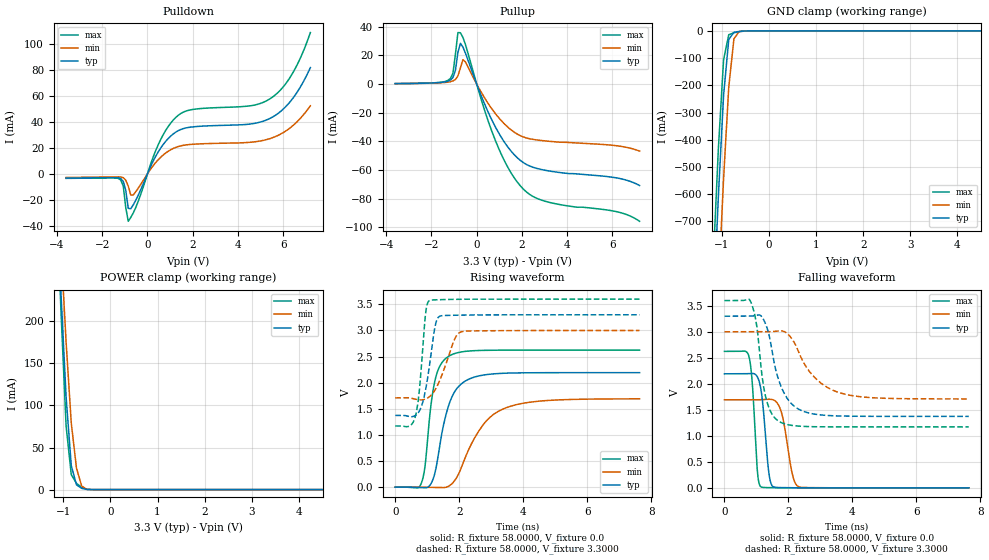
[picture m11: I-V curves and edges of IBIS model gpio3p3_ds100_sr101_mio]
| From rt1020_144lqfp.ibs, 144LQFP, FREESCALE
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[Model] gpio3p3_ds100_sr101_mio
|   Model gpio3p3_ds100_sr101_mio
| This model was characterised for following simulation conditions:
| External (pad) voltage:
|   - Typ: 3.3V,   - Min: 3.0V,   - Max: 3.6V
| Library cells for typ/min/max conditions are connected as defined below:
|  pad - External Pad
|  ipp_do - Core Input
|  ipp_obe - Output Buffer Enable
|  esd_boost - ovdd
|  ipp_dse0 - vssi
|  ipp_dse1 - vssi
|  ipp_dse2 - vddi
|  ipp_fsel0 - vddi
|  ipp_fsel1 - vssi
|  ipp_ina - ipp_ina
|  ipp_ind - ipp_ind
|  ipp_pwr_stable - vddi
|  ipp_sre - vddi
|  ovdd - ovdd
|  ovss - ovss
|  vddi - vddi
|  vssi - vssi
| All other pins connected to ground
Model_type I/O
Polarity   Non-Inverting
Enable   Active-High
Vinl =   0.9900V
Vinh =   2.3100V
Vmeas =  1.6500V
Cref =   0.0F
Rref =   58.0000
Vref =   1.6500V
C_comp   1.2178pF   1.1833pF   1.2636pF
|C_comp_pullup   0.6042pF   0.6189pF   0.5908pF
|C_comp_pulldown   0.5474pF   0.5788pF   0.5258pF
[Model Spec]
| variable   typ   min   max
Vinh   2.3100V   2.1000V   2.5200V
Vinl   0.9900V   0.9000V   1.0800V
S_overshoot_high   3.3000V   3.0000V   3.6000V
S_overshoot_low   0.0V   0.0V   0.0V
Vmeas   1.6500V   1.5000V   1.8000V
Vref   1.6500V   1.5000V   1.8000V
Cref   0.0F   0.0F   0.0F
Rref   58.0000   58.0000   58.0000
[Temperature Range]   25.0000   0.1050k   -20.0000
[Voltage Range]   3.3000V   3.0000V   3.6000V
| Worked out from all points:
|   slope of the pulldown table from 0 to 0.495 V, typ, clamps not added: 28.5 ohm
|   slope of the pullup table from 0 to 0.495 V, typ, clamps not added: 25.7 ohm
|   GND clamp passes 1 mA (typ) near -0.54 V on its own axis
|   POWER clamp passes 1 mA (typ) near -0.57 V on its own axis
|   rising waveform, R_fixture 58.0000, V_fixture 0.0: 20-80 % time 494ps typ, 946ps min, 310ps max; typ from 0 V to 2.19 V
|   rising waveform, R_fixture 58.0000, V_fixture 3.3000: 20-80 % time 287ps typ, 458ps min, 198ps max; typ from 1.37 V to 3.3 V
|   falling waveform, R_fixture 58.0000, V_fixture 0.0: 20-80 % time 187ps typ, 274ps min, 146ps max; typ from 2.19 V to 0 V
|   falling waveform, R_fixture 58.0000, V_fixture 3.3000: 20-80 % time 517ps typ, 894ps min, 318ps max; typ from 3.3 V to 1.37 V
[Pulldown]
|Voltage   I(typ)   I(min)   I(max)
-3.6V     -3.29mA    -2.84mA    -3.51mA
-1.18V    -3.645mA   -2.421mA   -4.835mA
-1.07V    -5.921mA   -3.024mA   -9.452mA
-960mV    -12.77mA   -4.911mA   -25.98mA
-850mV    -26.55mA   -9.409mA   -36.48mA
-630mV    -23.88mA   -16.25mA   -30.12mA
470mV     16.68mA    10.72mA    22.13mA
1.24V     31.86mA    20.19mA    43.07mA
1.9V      35.79mA    22.52mA    49.06mA
5.42V     42.57mA    27.03mA    57.6mA
6.3V      55.19mA    35.19mA    73.91mA
7.2V      81.51mA    52.18mA    108.4mA
[Pullup]
|Voltage   I(typ)   I(min)   I(max)
-3.6V     330uA      290uA      330uA
-1.27V    2.011mA    1.347mA    2.56mA
-1.05V    4.628mA    2.191mA    7.616mA
-940mV    9.591mA    3.262mA    21.02mA
-830mV    22.24mA    5.683mA    36mA
-720mV    28.46mA    11.34mA    35.87mA
-610mV    25.92mA    17.01mA    32.61mA
-500mV    21.74mA    15.5mA     27.75mA
820mV     -29.79mA   -20.52mA   -39.2mA
2.03V     -54.53mA   -36.77mA   -72.89mA
3.02V     -60.23mA   -39.71mA   -81.88mA
7.2V      -70.9mA    -46.86mA   -95.92mA
[GND_clamp]
|Voltage   I(typ)   I(min)   I(max)
-3.6V     -10.99A    -11.14A    -10.93A
-1.18V    -1.033A    -1.378A    -850.8mA
-1.07V    -607mA     -947.1mA   -431.4mA
-960mV    -236.8mA   -543mA     -106.4mA
-850mV    -31.63mA   -206.7mA   -14.18mA
-740mV    -5.424mA   -29mA      -7.092mA
-630mV    -2.275mA   -2.653mA   -3.283mA
-410mV    -62.05uA   -83.52uA   -82.05uA
7.2V      0A         0A         0A
[POWER_clamp]
|Voltage   I(typ)   I(min)   I(max)
-3.6V     3.491A     3.319A     3.949A
-1.16V    368.2mA    410.8mA    372.9mA
-1.05V    234.5mA    290.2mA    214.3mA
-940mV    110.2mA    175.6mA    75.85mA
-830mV    28.53mA    79.02mA    17.73mA
-720mV    5.671mA    25.66mA    7.515mA
-610mV    1.49mA     4.301mA    2.636mA
-500mV    198.2uA    300.8uA    424.4uA
-390mV    9.667uA    18.86uA    16.14uA
7.2V      0A         0A         0A
[Ramp]
| variable   typ   min   max
dV/dt_r  1.3153/0.4943n   1.0146/0.9461n   1.5740/0.3100n
dV/dt_f  1.1558/0.5174n   0.7745/0.8935n   1.4570/0.3177n
R_load = 58.0000
[Rising Waveform]
R_fixture= 58.0000
V_fixture= 0.0
V_fixture_min= 0.0
V_fixture_max= 0.0
|time   V(typ)   V(min)   V(max)
0s        4.578nV    4.118nV    48.47nV
812.4ps   -7.352mV   -280.5uV   70.58mV
927.4ps   -11.37mV   -1.371mV   386.3mV
1.095ns   45.7mV     -3.155mV   1.464V
1.238ns   263.5mV    -5.322mV   2.032V
1.687ns   1.595V     24.49mV    2.512V
2.225ns   2.045V     621.1mV    2.602V
2.792ns   2.15V      1.228V     2.62V
3.305ns   2.178V     1.478V     2.623V
7.64ns    2.192V     1.691V     2.623V
[Rising Waveform]
R_fixture= 58.0000
V_fixture= 3.3000
V_fixture_min= 3.0000
V_fixture_max= 3.6000
|time   V(typ)   V(min)   V(max)
0s        1.374V     1.709V     1.172V
632.7ps   1.374V     1.684V     1.364V
748.4ps   1.453V     1.672V     1.825V
956.2ps   1.89V      1.69V      3.362V
1.07ns    2.326V     1.732V     3.573V
1.225ns   3.012V     1.842V     3.586V
1.333ns   3.241V     1.965V     3.588V
1.84ns    3.291V     2.813V     3.596V
2.079ns   3.294V     2.978V     3.598V
7.64ns    3.3V       3V         3.6V
[Falling Waveform]
R_fixture= 58.0000
V_fixture= 0.0
V_fixture_min= 0.0
V_fixture_max= 0.0
|time   V(typ)   V(min)   V(max)
0s        2.192V     1.692V     2.623V
770.4ps   2.197V     1.691V     2.514V
876.7ps   2.199V     1.692V     1.954V
1.033ns   2.127V     1.692V     290.3mV
1.151ns   1.852V     1.695V     16.71mV
1.392ns   268.7mV    1.703V     4.273mV
1.53ns    19.49mV    1.69V      2.918mV
1.777ns   4.84mV     1.459V     1.55mV
2.313ns   1.546mV    23.87mV    388.3uV
7.64ns    943nV      4.223uV    325.8nV
[Falling Waveform]
R_fixture= 58.0000
V_fixture= 3.3000
V_fixture_min= 3.0000
V_fixture_max= 3.6000
|time   V(typ)   V(min)   V(max)
0s        3.3V       3V         3.6V
821.2ps   3.3V       3V         3.575V
993.7ps   3.316V     3V         3.175V
1.179ns   3.278V     2.999V     2.13V
1.293ns   3.138V     2.999V     1.735V
1.742ns   1.991V     3.018V     1.264V
2.298ns   1.52V      2.645V     1.188V
2.808ns   1.418V     2.129V     1.175V
3.503ns   1.383V     1.848V     1.172V
7.64ns    1.374V     1.709V     1.172V
